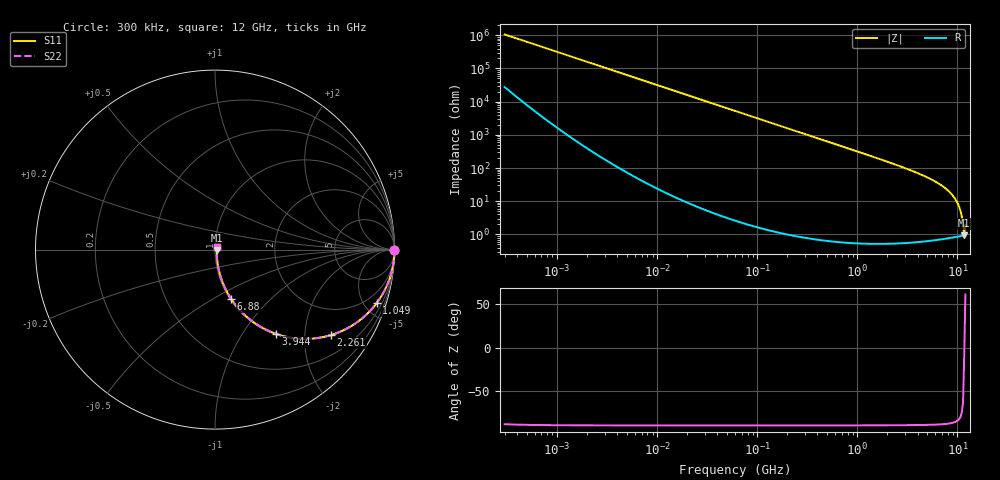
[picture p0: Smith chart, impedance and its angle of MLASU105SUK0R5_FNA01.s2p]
! MLASU105SUK0R5_FNA01  S-PARAMETER MODEL  ( General Type )
! Model Generated by TAIYO YUDEN Corporation (http://www.ty-top.com)
! Version 2.0
! TAIYO YUDEN Control No. 120810
! Copyright(c) 2011 TAIYO YUDEN CO.,LTD. All Rights Reserved.
! Product Description (link to TY-COMPAS)
! https://ds.yuden.co.jp/TYCOMPAS/or/detail?pn=MLASU105SUK0R5CFNA01&u=M
! Products Name : Multilayer Ceramic Capacitors
! Characteristics :
!  Capacitance : 0.5 pF , Rated Voltage : 50V , TCC : UK / U2K
!  Case Size : 1.0 x 0.5 / 0.039 x 0.02 [mm/inch] , Thickness : 0.5 / 0.02 [mm/inch]
!  (Conditions: Temperature = 25 degC , DC Bias Current/Voltage = 0A / 0V)
! External Node Assignments :
!  1  o---| |---o  2
! GND o---------o GND
! Frequency Range : 0.3MHz  -  12000MHz  [ 401 STEP ]
# MHz S RI R 50
! Freq[MHz].  S11 Real  S11 Imag  S21 Real  S21 Imag  S12 Real  S12 Imag  S22 Real  S22 Imag
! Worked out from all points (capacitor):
!   401 points, 300 kHz to 12 GHz, reference 50 ohm
!   read as one part in series: C = 501 fF near 316.3 kHz
!   lowest |Z| = 939 mohm at 11.69 GHz (marker M1)
!   series resonance near 11.71 GHz, so ESL is about 370 pH
!   S11 on the Smith chart (normalised r, x): 300 kHz: open; 1.049 GHz: 1.01, -6.01; 2.261 GHz: 1.01, -2.71; 3.944 GHz: 1.01, -1.43; 6.88 GHz: 1.01, -0.61; 12 GHz: 1.02, +0.03
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0.3  1 -9.44e-05  2.47e-06 9.44e-05  2.47e-06 9.44e-05  1 -9.44e-05
0.342489  1 -0.000108  2.31e-06 0.000108  2.31e-06 0.000108  1 -0.000108
1.769972  1 -0.000557  1.86e-06 0.000557  1.86e-06 0.000557  1 -0.000557
10.44266  1 -0.00329  1.32e-05 0.00329  1.32e-05 0.00329  1 -0.00329
60  0.9996 -0.0189  0.000365 0.0189  0.000365 0.0189  0.9996 -0.0189
353.9943  0.9876 -0.1101  0.0124 0.1101  0.0124 0.1101  0.9876 -0.1101
668.5285  0.9571 -0.2019  0.0429 0.2019  0.0429 0.2019  0.9571 -0.2019
1048.836  0.9 -0.2992  0.1 0.2992  0.1 0.2992  0.9 -0.2992
1480.043  0.8165 -0.3859  0.1835 0.3859  0.1835 0.3859  0.8165 -0.3859
2088.533  0.6841 -0.4631  0.3159 0.4631  0.3159 0.4631  0.6841 -0.4631
2261.293  0.6464 -0.4762  0.3536 0.4762  0.3536 0.4762  0.6464 -0.4762
3026.31  0.4903 -0.4971  0.5097 0.4971  0.5097 0.4971  0.4903 -0.4971
3944.255  0.3396 -0.4695  0.6604 0.4695  0.6604 0.4695  0.3396 -0.4695
5420.343  0.1791 -0.3765  0.8209 0.3765  0.8209 0.3765  0.1791 -0.3765
6879.757  0.0898 -0.2745  0.9102 0.2745  0.9102 0.2745  0.0898 -0.2745
8503.825  0.0378 -0.17  0.9622 0.17  0.9622 0.17  0.0378 -0.17
9708.23  0.0187 -0.1012  0.9813 0.1012  0.9813 0.1012  0.0187 -0.1012
10511.28  0.0122 -0.0592  0.9878 0.0592  0.9878 0.0592  0.0122 -0.0592
10793.46  0.0108 -0.0451  0.9892 0.0451  0.9892 0.0451  0.0108 -0.0451
11083.22  0.0099 -0.0311  0.9901 0.0311  0.9901 0.0311  0.0099 -0.0311
11686.27  0.00921 -0.00136  0.9908 0.00136  0.9908 0.00136  0.00921 -0.00136
12000  0.00963 0.0169  0.9904 -0.0169  0.9904 -0.0169  0.00963 0.0169
